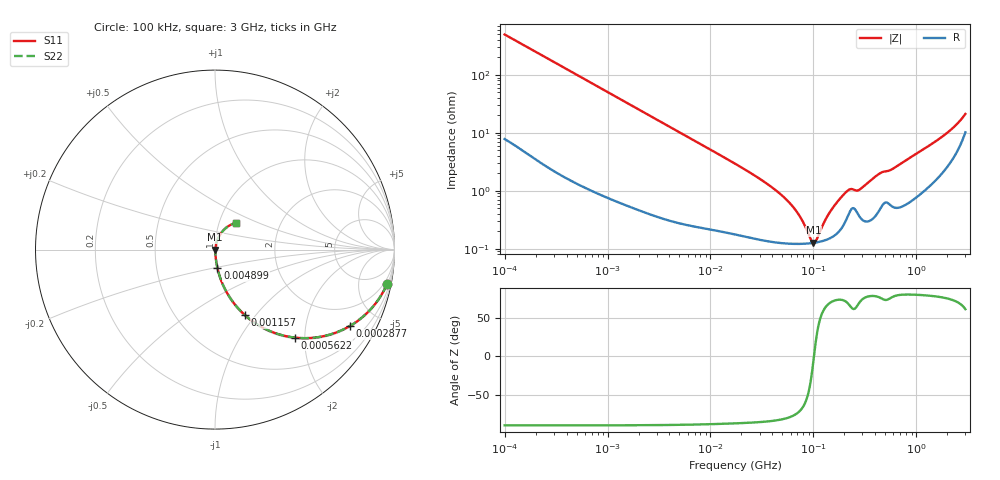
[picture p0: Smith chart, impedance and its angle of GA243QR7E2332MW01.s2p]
!Murata Part Number: GA243QR7E2332MW01
!These Parameters are Measured in Series Mode Connection
!Data Generated on Jun 19, 2026
!  o--ll--o
!Port1  Port2
!  o------o
!Operation Temp=25[degC], DC Bias Voltage=0[V]
!Freq. Start=100[kHz] Stop=3[GHz] 401[Steps]
# Hz S RI R 50
!Freq.(Hz) S11(Real) S11(Imag) S21(Real) S21(Imag) S12(Real) S12(Imag) S22(Real) S22(Imag)
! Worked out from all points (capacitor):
!   401 points, 100 kHz to 3 GHz, reference 50 ohm
!   read as one part in series: C = 3.19 nF near 105.3 kHz
!   lowest |Z| = 127 mohm at 99.92 MHz (marker M1)
!   series resonance near 101.3 MHz, so ESL is about 770 pH
!   S11 on the Smith chart (normalised r, x): 100 kHz: 1, -10; 287.7 kHz: 1.05, -3.49; 562.2 kHz: 1.02, -1.80; 1.157 MHz: 1.01, -0.88; 4.899 MHz: 1.01, -0.21; 3 GHz: 1.20, +0.37
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100000  0.9584 -0.192  0.0416 0.192  0.0416 0.192  0.9584 -0.192
176296  0.8863 -0.3104  0.1137 0.3104  0.1137 0.3104  0.8863 -0.3104
287677  0.7504 -0.4263  0.2496 0.4263  0.2496 0.4263  0.7504 -0.4263
562235  0.447 -0.4906  0.553 0.4906  0.553 0.4906  0.447 -0.4906
1156955  0.1651 -0.3636  0.8349 0.3636  0.8349 0.3636  0.1651 -0.3636
3161081  0.0287 -0.1565  0.9713 0.1565  0.9713 0.1565  0.0287 -0.1565
4899066  0.0135 -0.1029  0.9865 0.1029  0.9865 0.1029  0.0135 -0.1029
1.77727e7  0.00255 -0.0284  0.9974 0.0284  0.9974 0.0284  0.00255 -0.0284
3.564176e7  0.00152 -0.013  0.9985 0.013  0.9985 0.013  0.00152 -0.013
5.523785e7  0.00127 -0.00679  0.9987 0.00679  0.9987 0.00679  0.00127 -0.00679
7.334282e7  0.00122 -0.00348  0.9988 0.00348  0.9988 0.00348  0.00122 -0.00348
9.738194e7  0.00125 -0.00042  0.9988 0.00042  0.9988 0.00042  0.00125 -0.00042
9.992433e7  0.00126 -0.000144  0.9987 0.000144  0.9987 0.000144  0.00126 -0.000144
1.079567e8  0.00129 0.000686  0.9987 -0.000686  0.9987 -0.000686  0.00129 0.000686
1.470833e8  0.00155 0.0042  0.9985 -0.0042  0.9985 -0.0042  0.00155 0.0042
2.056221e8  0.00306 0.00878  0.9969 -0.00878  0.9969 -0.00878  0.00306 0.00878
2.279507e8  0.00454 0.00958  0.9955 -0.00958  0.9955 -0.00958  0.00454 0.00958
2.801453e8  0.00369 0.00972  0.9963 -0.00972  0.9963 -0.00972  0.00369 0.00972
4.341712e8  0.00482 0.0188  0.9952 -0.0188  0.9952 -0.0188  0.00482 0.0188
5.475153e8  0.00627 0.0213  0.9937 -0.0213  0.9937 -0.0213  0.00627 0.0213
1.701687e9  0.0237 0.0753  0.9763 -0.0753  0.9763 -0.0753  0.0237 0.0753
3e9  0.1176 0.1486  0.8824 -0.1486  0.8824 -0.1486  0.1176 0.1486
